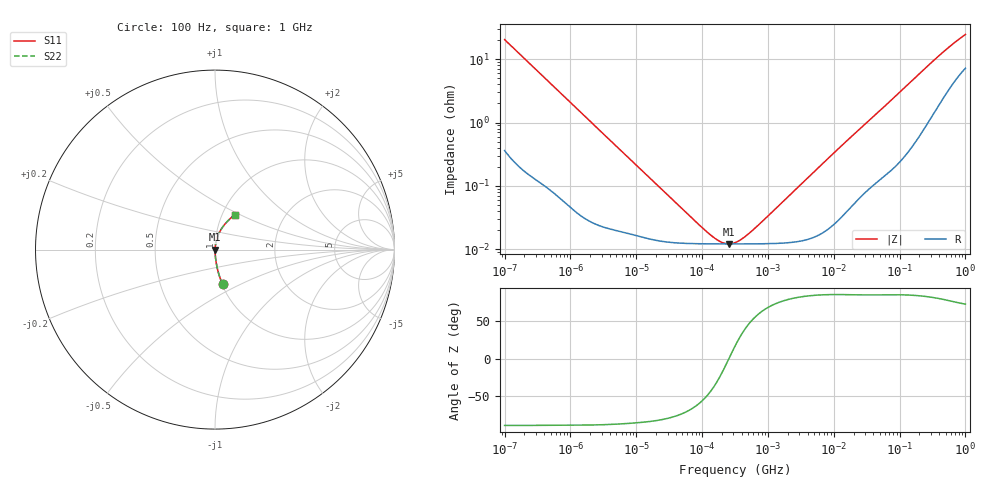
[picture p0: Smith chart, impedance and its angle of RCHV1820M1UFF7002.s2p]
! RCHV1820M1UFF7002  S-PARAMETER MODEL  (AEC-Q200 qualified)
! Model Generated by ELNA Corporation (http://www.ty-top.com)
! Version 1.0
! ELNA Control No. 240229
! Copyright (c) 2024 ELNA CO.,LTD. All Rights Reserved.
! Products Name : CONDUCTIVE POLYMER HYBRID ALUMINUM ELECTROLYTIC CAPACITORS
! Characteristics :
!  Capacitance  :  82uF  ,  Rated voltage  :  50V
!  Operating Temp. Range  :  -55 to +105 degC  ,  Endurance  :  5000hr at 105 degC
!  Dimension D  :  10mm  ,  Dimension L  :  8.7mm
! Frequency Range : 100Hz - 1GHz
! External Node Assignments :
!  1  o---| |---o  2
# MHz S RI R 50
!Freq[MHz].  S11 Real  S11 Imag  S21 Real  S21 Imag  S12 Real  S12 Imag  S22 Real  S22 Imag
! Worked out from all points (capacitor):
!   401 points, 100 Hz to 1 GHz, reference 50 ohm
!   read as one part in series: C = 78.1 uF near 108 Hz
!   lowest |Z| = 12.2 mohm at 258.5 kHz (marker M1)
!   series resonance near 255.1 kHz, so ESL is about 5 nH
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0.0001  0.043 -0.1941  0.957 0.1941  0.957 0.1941  0.043 -0.1941
0.000113  0.0343 -0.1737  0.9657 0.1737  0.9657 0.1737  0.0343 -0.1737
0.000183  0.014 -0.1097  0.986 0.1097  0.986 0.1097  0.014 -0.1097
0.000309  0.00557 -0.0658  0.9944 0.0658  0.9944 0.0658  0.00557 -0.0658
0.000613  0.00184 -0.0336  0.9982 0.0336  0.9982 0.0336  0.00184 -0.0336
0.001488  0.000526 -0.014  0.9995 0.014  0.9995 0.014  0.000526 -0.014
0.022131  0.000137 -0.000966  0.9999 0.000966  0.9999 0.000966  0.000137 -0.000966
0.083657  0.000123 -0.000231  0.9999 0.000231  0.9999 0.000231  0.000123 -0.000231
0.135675  0.000122 -0.000115  0.9999 0.000115  0.9999 0.000115  0.000122 -0.000115
0.194984  0.000122 -4.62e-05  0.9999 4.62e-05  0.9999 4.62e-05  0.000122 -4.62e-05
0.229087  0.000122 -1.83e-05  0.9999 1.83e-05  0.9999 1.83e-05  0.000122 -1.83e-05
0.258523  0.000122 2.33e-06  0.9999 -2.33e-06  0.9999 -2.33e-06  0.000122 2.33e-06
0.316228  0.000122 3.69e-05  0.9999 -3.69e-05  0.9999 -3.69e-05  0.000122 3.69e-05
0.419276  0.000122 8.81e-05  0.9999 -8.81e-05  0.9999 -8.81e-05  0.000122 8.81e-05
0.60256  0.000122 0.000165  0.9999 -0.000165  0.9999 -0.000165  0.000122 0.000165
4.704354  0.000154 0.00156  0.9998 -0.00156  0.9998 -0.00156  0.000154 0.00156
15.13561  0.000401 0.00493  0.9996 -0.00493  0.9996 -0.00493  0.000401 0.00493
69.9842  0.0021 0.021  0.9979 -0.021  0.9979 -0.021  0.0021 0.021
176.8072  0.00767 0.0514  0.9923 -0.0514  0.9923 -0.0514  0.00767 0.0514
395.8221  0.0301 0.1061  0.9699 -0.1061  0.9699 -0.1061  0.0301 0.1061
668.3439  0.0671 0.1554  0.9329 -0.1554  0.9329 -0.1554  0.0671 0.1554
1000  0.1096 0.1946  0.8904 -0.1946  0.8904 -0.1946  0.1096 0.1946
